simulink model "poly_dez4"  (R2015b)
settings: Solver=VariableStepAuto  StartTime=0.0  StopTime=15  RelTol=1e-3
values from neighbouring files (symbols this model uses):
  g = firpolyphase(hdez, M)    [poly_dez_1.m]    (also in poly_dez_2.m; poly_interp_1.m = firpolyphase(hint, L); poly_interp_2.m = firpolyphase(hint, L))
undefined symbols (not defined in the file or in its folder): fir1
libraries: simulink x1, dspbuff3 x1, dspmlti4 x1

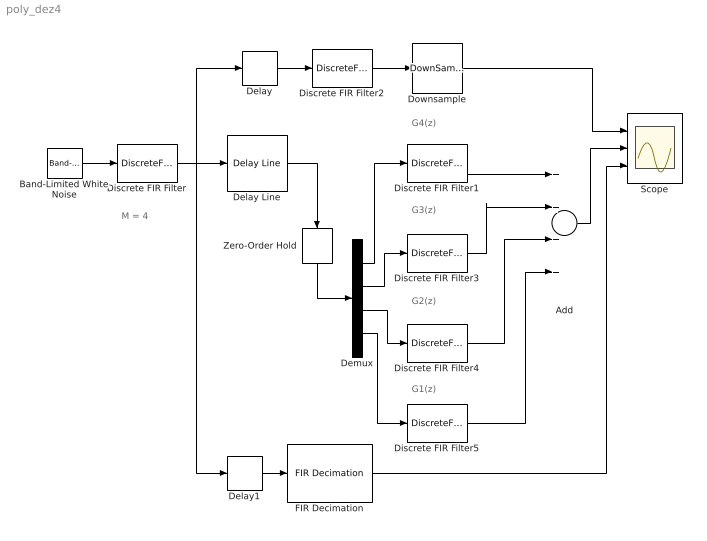
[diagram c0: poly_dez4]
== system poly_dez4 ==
  note: G1(z)
  note: G2(z)
  note: G3(z)
  note: G4(z)
  note: M = 4
  Add : Sum  Inputs=++++
  Band-Limited White Noise : simulink/Sources/Band-Limited White Noise  Cov=[0.1]  Ts=0.1  seed=[23341]
  Delay : Delay  DelayLength=1
  Delay Line : dspbuff3/Delay Line  siz=4  ic=0  directfeed=off  enable_output=off  hold_output=off  TreatMby1Signals=One channel  OutputFrames=off
  Delay1 : Delay  DelayLength=1
  Demux : Demux
  Discrete FIR Filter : DiscreteFir  Coefficients=fir1(128, 0.2)
  Discrete FIR Filter1 : DiscreteFir  Coefficients=(g(4,:))
  Discrete FIR Filter2 : DiscreteFir  Coefficients=fir1(32,1/4)
  Discrete FIR Filter3 : DiscreteFir  Coefficients=(g(3,:))
  Discrete FIR Filter4 : DiscreteFir  Coefficients=(g(2,:))
  Discrete FIR Filter5 : DiscreteFir  Coefficients=(g(1,:))
  Downsample : DownSample  N=4  RateOptions=Allow multirate processing
  FIR Decimation : dspmlti4/FIR Decimation  FilterSource=Dialog parameters  h=hdez  D=4  filtStruct=Direct form  FilterObject=FDECIM  InputProcessing=Columns as channels (frame based)  framing=Allow multirate processing  inputOffset=0  outputBufInitCond=0  roundingMode=Floor  overflowMode=off  firstCoeffDataTypeStr=Inherit: Same word length as input  firstCoeffMin=[]  firstCoeffMax=[]  firstCoeffLastDataTypeStr=Inherit: Same word length as input  outputDataTypeStr=Inherit: Same as accumulator  outputMin=[]  outputMax=[]  outputLastDataTypeStr=Inherit: Same as accumulator
  Scope : Scope  NumInputPorts=3
  Zero-Order Hold : ZeroOrderHold  SampleTime=0.1*4
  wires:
  Band-Limited White Noise/1 -> Discrete FIR Filter/1
  Discrete FIR Filter1/1 -> Add/1
  Discrete FIR Filter3/1 -> Add/2
  Discrete FIR Filter4/1 -> Add/3
  Add/1 -> Scope/2
  Discrete FIR Filter5/1 -> Add/4
  Downsample/1 -> Scope/1
  Discrete FIR Filter/1 -> Delay1/1, Delay Line/1, Delay/1
  Demux/4 -> Discrete FIR Filter5/1
  Demux/1 -> Discrete FIR Filter1/1
  Demux/3 -> Discrete FIR Filter4/1
  Demux/2 -> Discrete FIR Filter3/1
  Zero-Order Hold/1 -> Demux/1
  Discrete FIR Filter2/1 -> Downsample/1
  Delay/1 -> Discrete FIR Filter2/1
  Delay Line/1 -> Zero-Order Hold/1
  FIR Decimation/1 -> Scope/3
  Delay1/1 -> FIR Decimation/1
